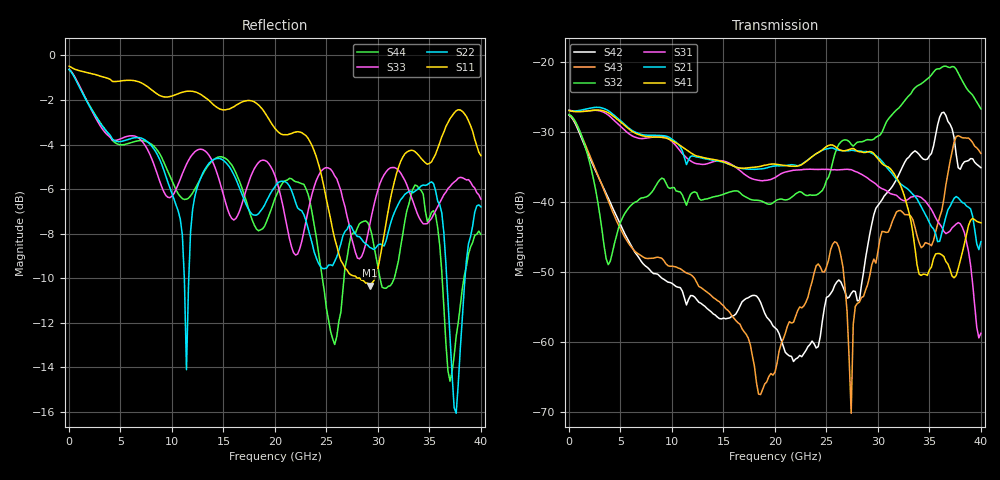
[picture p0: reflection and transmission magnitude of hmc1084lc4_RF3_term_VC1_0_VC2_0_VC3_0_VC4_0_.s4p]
!Agilent Technologies,N5224A,MY51441122,A.09.40.06
!Agilent N5224A: A.09.40.06
!Date: Thursday, June 19, 2014 00:52:02
!Correction: S11(Full 4 Port(1,2,3,4))
!S12(Full 4 Port(1,2,3,4))
!S13(Full 4 Port(1,2,3,4))
!S14(Full 4 Port(1,2,3,4))
!S21(Full 4 Port(1,2,3,4))
!S22(Full 4 Port(1,2,3,4))
!S23(Full 4 Port(1,2,3,4))
!S24(Full 4 Port(1,2,3,4))
!S31(Full 4 Port(1,2,3,4))
!S32(Full 4 Port(1,2,3,4))
!S33(Full 4 Port(1,2,3,4))
!S34(Full 4 Port(1,2,3,4))
!S41(Full 4 Port(1,2,3,4))
!S42(Full 4 Port(1,2,3,4))
!S43(Full 4 Port(1,2,3,4))
!S44(Full 4 Port(1,2,3,4))
!S4P File: Measurements: <S11,S12,S13,S14>,
!<S21,S22,S23,S24>,
!<S31,S32,S33,S34>,
!<S41,S42,S43,S44>:
# Hz S  dB  R 50
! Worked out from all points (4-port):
!   201 points, 10 MHz to 40 GHz, reference 50 ohm
!   strongest paths, dB at 10 MHz, 10.01 GHz, 20 GHz, 30 GHz, 40 GHz:
!     S41: -27.0, -31.3, -34.6, -33.8, -43.0
!     S21: -26.9, -31.1, -34.9, -33.6, -45.7
!     S31: -26.9, -31.4, -36.5, -37.7, -58.7
!     S32: -27.5, -37.9, -39.9, -30.6, -26.7
!     S43: -27.5, -49.2, -64.3, -47.1, -33.1
!     S42: -27.6, -51.6, -57.9, -40.5, -35.1
!   lowest |S11| = -10.3 dB at 29.2 GHz (marker M1), VSWR 1.88, Z = 77 + j29.1 ohm
!   |S11| at or under -10 dB: 28.24 GHz to 29.68 GHz (1.442 GHz wide, 4.98 % of centre)
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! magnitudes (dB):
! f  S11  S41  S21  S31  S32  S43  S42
! 10 MHz  -0.5  -27.0  -26.9  -26.9  -27.5  -27.5  -27.6
! 3.809 GHz  -1.0  -27.3  -27.0  -27.6  -48.9  -39.8  -39.4
! 18.81 GHz  -2.4  -34.8  -35.3  -37.0  -39.9  -66.7  -55.1
! 25.8 GHz  -8.2  -32.0  -32.4  -35.4  -33.2  -45.7  -51.9
! 27.4 GHz  -9.9  -32.4  -32.6  -35.4  -31.7  -70.1  -53.0
! 29.2 GHz  -10.3  -32.8  -32.9  -36.8  -31.1  -50.5  -44.6
! 40 GHz  -4.5  -43.0  -45.7  -58.7  -26.7  -33.1  -35.1
